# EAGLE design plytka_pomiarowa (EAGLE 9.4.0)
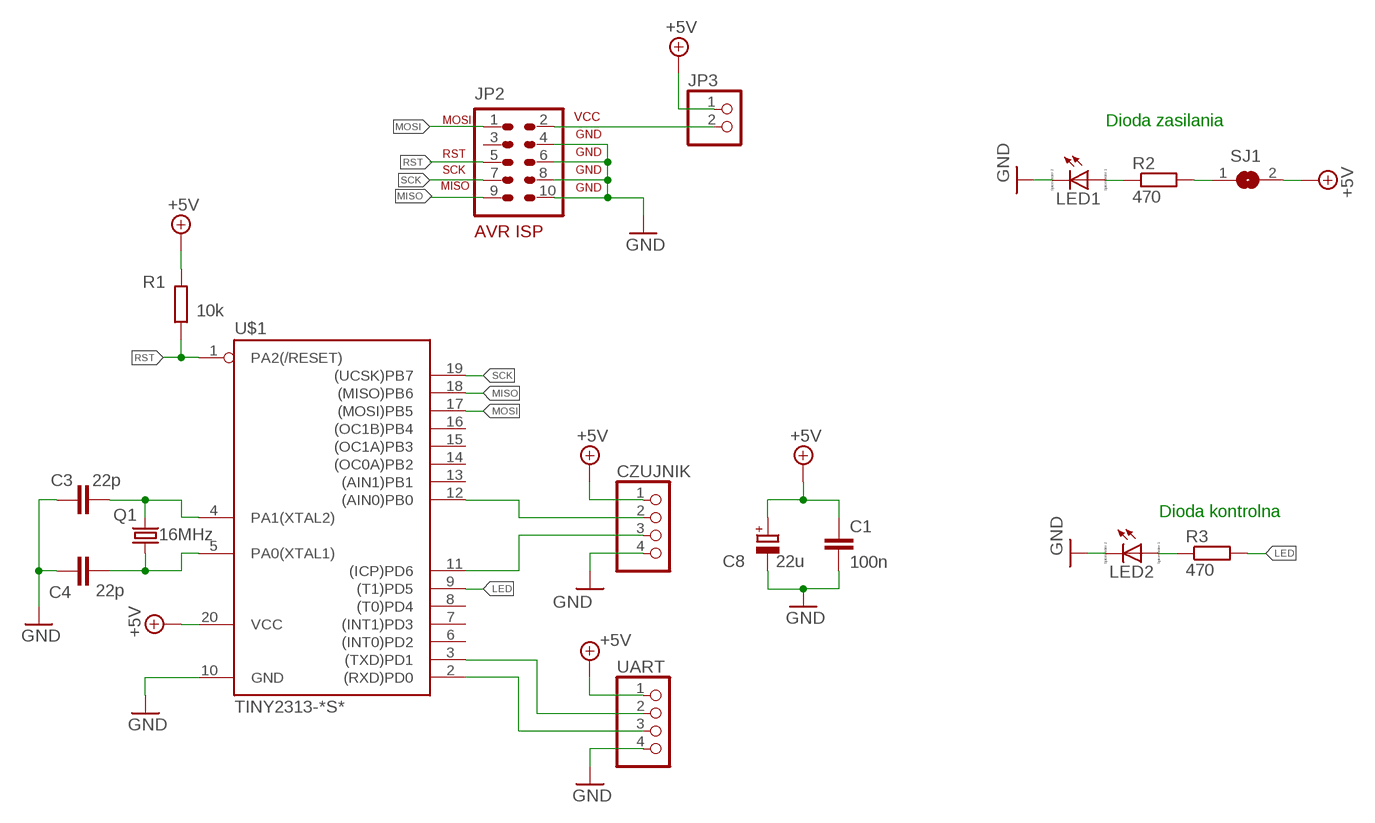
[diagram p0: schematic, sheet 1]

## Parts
C1  100n  C-EUC1206  [C1206]
C3  22p  C-EUC1206  [C1206]
C4  22p  C-EUC1206  [C1206]
C8  22u  CPOL-EUSMCB  [SMC_B]
CZUJNIK  PINHD-1X4  [1X04]
JP2  AVR-ISP-10  [AVR-ISP-10]
JP3  PINHD-1X2  [1X02]
LED1  LED_E  [LED_1206]
LED2  LED_E  [LED_1206]
Q1  16MHz  KX-KS  [11.4X4.5]
R1  10k  R-EU_M1206  [M1206]
R2  470  R-EU_M1206  [M1206]
R3  470  R-EU_M1206  [M1206]
SJ1  SJ  [SJ]
U$1  TINY2313-*S*  [SO20L$]
UART  PINHD-1X4  [1X04]

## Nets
+5V: C1.1 C8.+ CZUJNIK.1 JP3.1 R1.2 SJ1.2 U$1.20(VCC) UART.1
ECHO: CZUJNIK.3 U$1.11((ICP)PD6)
GND: C1.2 C3.1 C4.1 C8.- CZUJNIK.4 JP2.4 JP2.6 JP2.8 JP2.10 LED1.C LED2.C U$1.10(GND) UART.4
LED: R3.2 U$1.9((T1)PD5)
MISO: JP2.9 U$1.18((MISO)PB6)
MOSI: JP2.1 U$1.17((MOSI)PB5)
N$1: C3.2 Q1.2 U$1.4(PA1(XTAL2))
N$2: C4.2 Q1.1 U$1.5(PA0(XTAL1))
N$3: JP2.2 JP3.2
N$4: R2.2 SJ1.1
N$5: LED1.A R2.1
N$7: LED2.A R3.1
RST: JP2.5 R1.1 U$1.1(PA2(/RESET))
RX: U$1.2((RXD)PD0) UART.3
SCK: JP2.7 U$1.19((UCSK)PB7)
TRIG: CZUJNIK.2 U$1.12((AIN0)PB0)
TX: U$1.3((TXD)PD1) UART.2
Unconnected: JP2.3 U$1.6((INT0)PD2) U$1.7((INT1)PD3) U$1.8((T0)PD4) U$1.13((AIN1)PB1) U$1.14((OC0A)PB2) U$1.15((OC1A)PB3) U$1.16((OC1B)PB4)

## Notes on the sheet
- Dioda zasilania
- Dioda kontrolna

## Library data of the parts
C1 C3 C4 = resistor:C-EU: CAPACITOR, European symbol
C8 = resistor:CPOL-EU: POLARIZED CAPACITOR, European symbol
CZUJNIK = pinhead:PINHD-1X4: PIN HEADER
JP2 = avr-7:AVR-ISP-10: AVR ISP-10 Serial Programming Header
JP3 = pinhead:PINHD-1X2: PIN HEADER
LED1 LED2 = eagle-ltspice:LED_E: LED; SPICEMODEL: NONE; SPICEPREFIX: D; SPICETYPE: diode
Q1 = crystal-geyer_V1_0:KX
R1-R3 = resistor:R-EU_: RESISTOR, European symbol
SJ1 = jumper:SJ: SMD solder JUMPER
U$1 = avr-7:TINY2313*: Atmel Tiny2313 2K Flash, 128 bytes EEPROM, 128 bytes RAM
UART = pinhead:PINHD-1X4: PIN HEADER; SPICEPREFIX: E

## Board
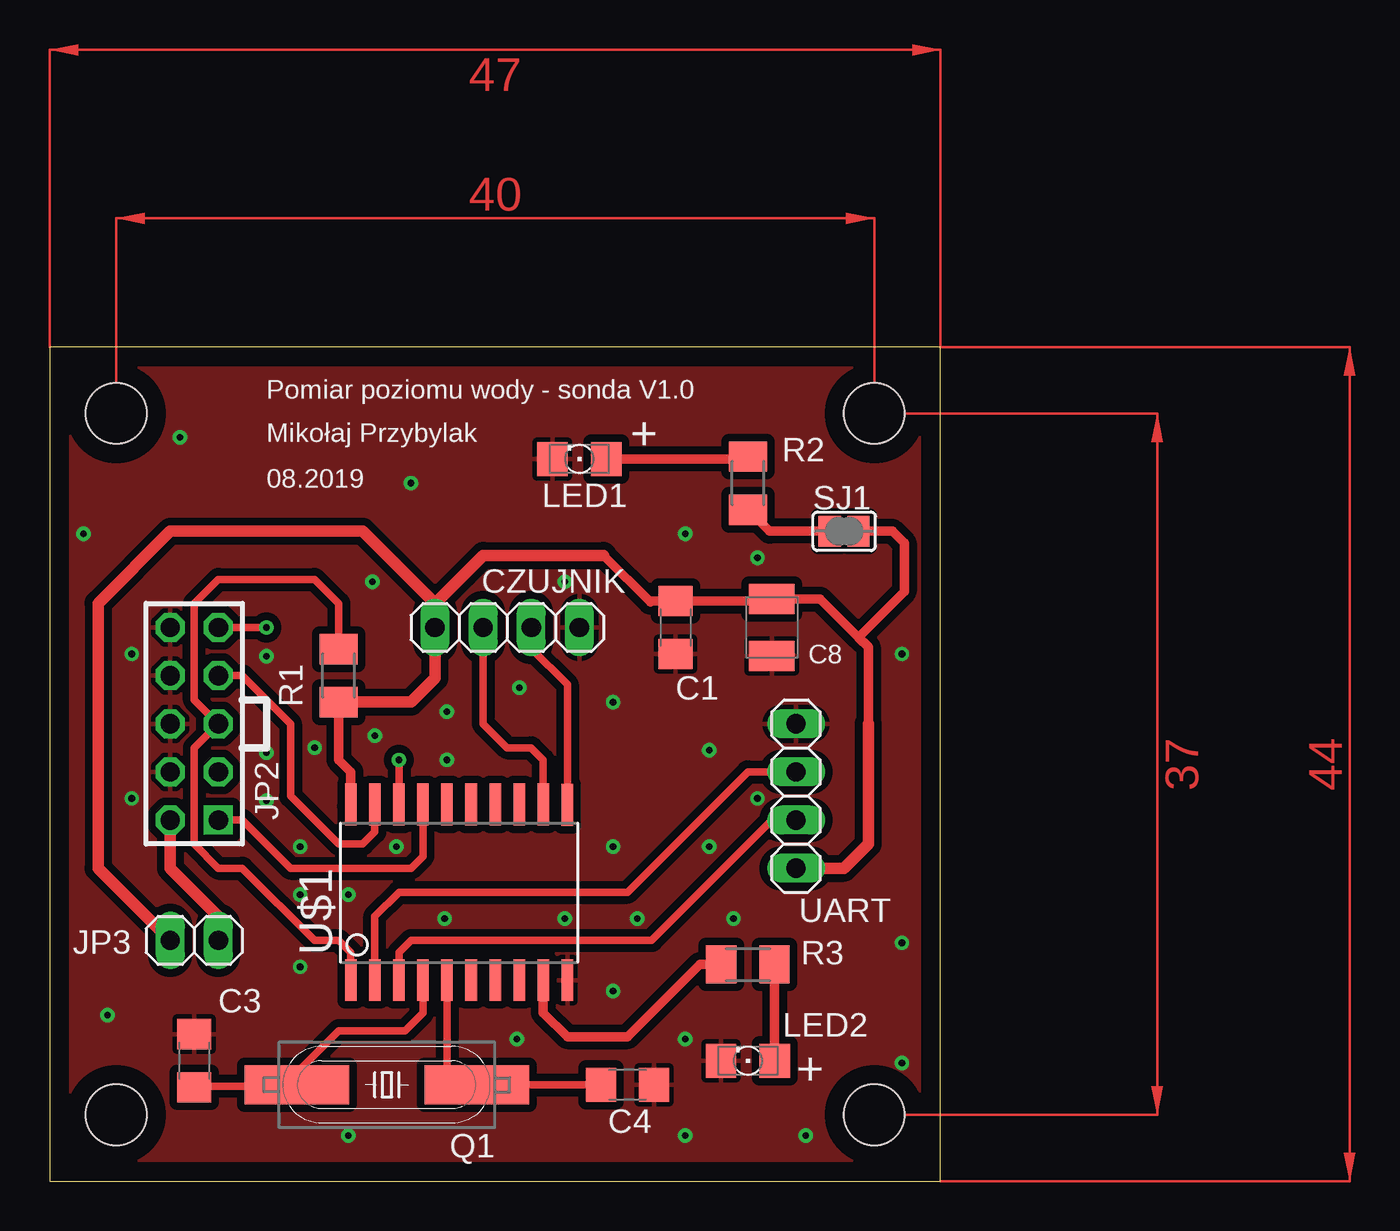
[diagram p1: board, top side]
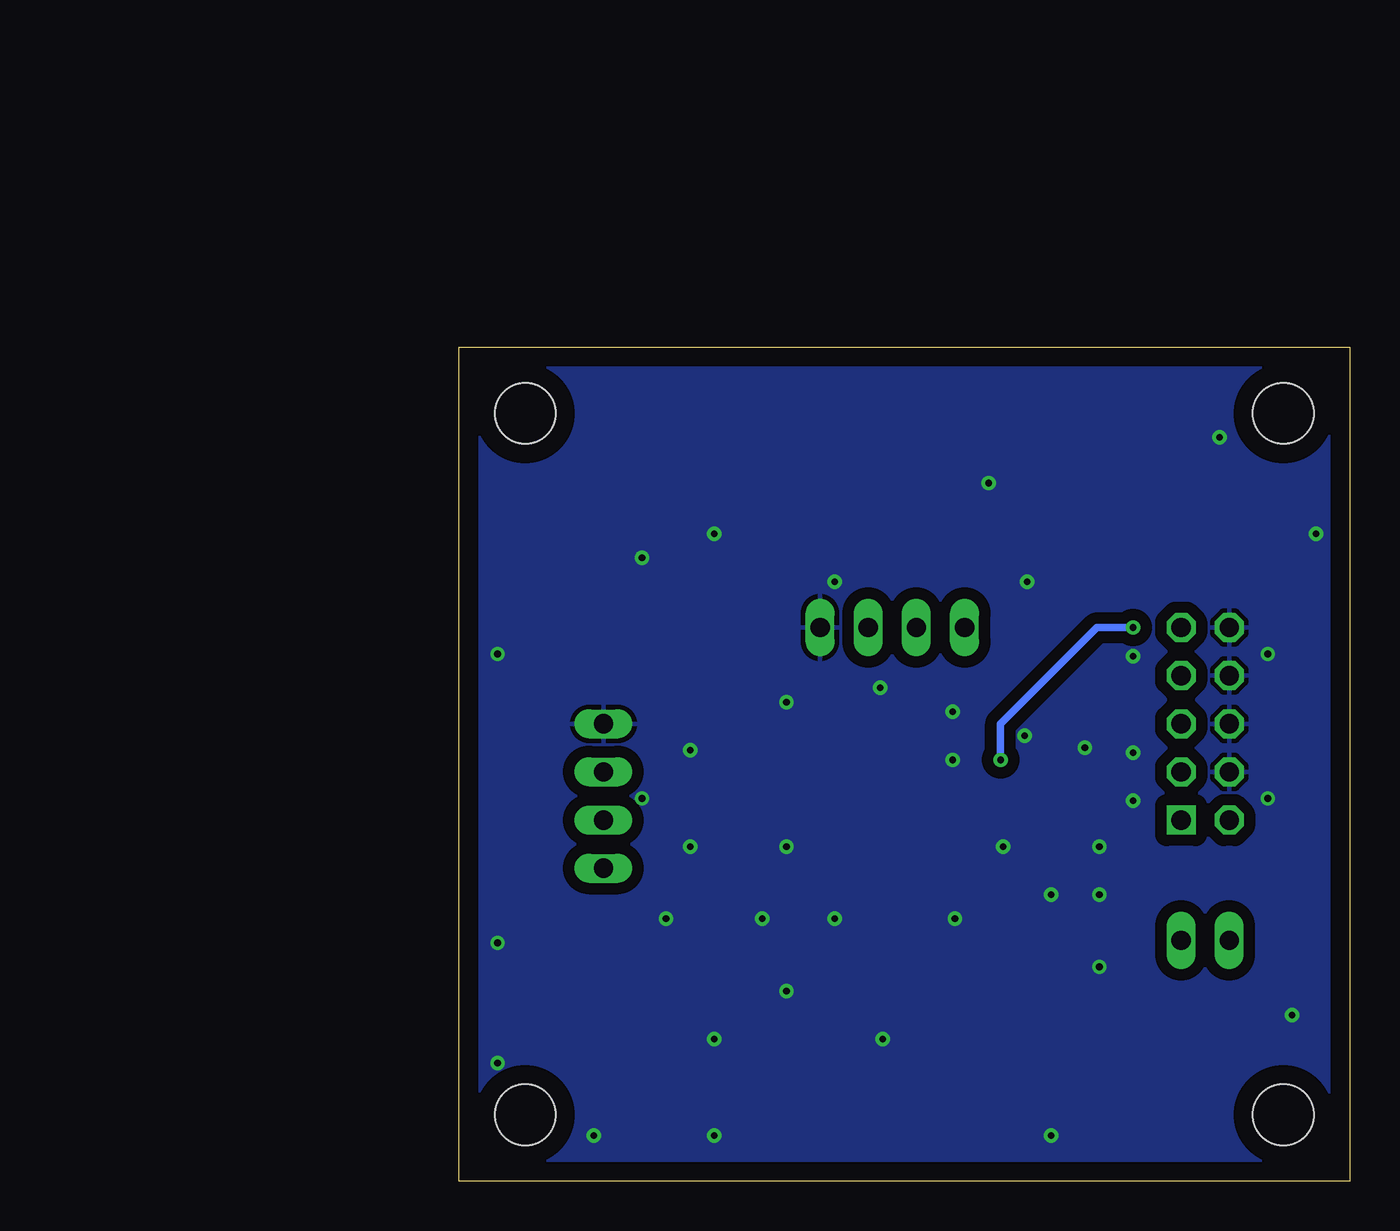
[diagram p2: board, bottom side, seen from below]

Size 47 x 44 mm. Coordinates in mm from the lower left corner, seen from the top.
Outline: 0,0 47,0 47,44 0,44 0,0
Copper layers (1*16): Top 0.035mm / dielectric 1.5mm / Bottom 0.035mm
Design rules "default *": minimum track width 6mil, minimum drill 0.5mm, track to track 10mil, track to pad 10mil, pad to pad 10mil, via to via 10mil, smd to smd 6mil, copper to edge 40mil, drill to drill 6mil, minimum pad ring 10mil, minimum via ring 8mil, stop-mask expansion 4mil, vias tented up to drill 0mil, thermal gap 10mil
Holes 3.2 mm at 3.5,40.5 43.5,40.5 43.5,3.5 3.5,3.5

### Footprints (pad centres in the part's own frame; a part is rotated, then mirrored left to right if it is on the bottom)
C1206 = smd 1.6 x 1.8: 1 -1.4,0; 2 1.4,0
SMC_B = smd 1.6 x 2.4: + -1.5,0; - 1.5,0
1X04 = drill 1.016 long: 1 -3.81,0; 2 -1.27,0; 3 1.27,0; 4 3.81,0
AVR-ISP-10 = drill 1.016 square: 1 -5.08,-1.27 | drill 1.016 octagon: 2 -5.08,1.27; 3 -2.54,-1.27; 4 -2.54,1.27; 5 0,-1.27; 6 0,1.27; 7 2.54,-1.27; 8 2.54,1.27; 9 5.08,-1.27; 10 5.08,1.27
1X02 = drill 1.016 long: 1 -1.27,0; 2 1.27,0
LED_1206 = smd 1.6 x 1.803: A -1.422,0; C 1.422,0
11.4X4.5 = smd 5.5 x 2.08: 1 -4.75,0; 2 4.75,0
M1206 = smd 1.6 x 2: 1 -1.4,0; 2 1.4,0
SJ = smd 1.168 x 1.6: 1 -0.762,0; 2 0.762,0
SO20L$ = smd 0.61 x 2.21: 1 -5.715,-4.636; 2 -4.445,-4.636; 3 -3.175,-4.636; 4 -1.905,-4.636; 5 -0.635,-4.636; 6 0.635,-4.636; 7 1.905,-4.636; 8 3.175,-4.636; 9 4.445,-4.636; 10 5.715,-4.636; 11 5.715,4.61; 12 4.445,4.636; 13 3.175,4.636; 14 1.905,4.636; 15 0.635,4.636; 16 -0.635,4.636; 17 -1.905,4.636; 18 -3.175,4.636; 19 -4.445,4.636; 20 -5.715,4.636

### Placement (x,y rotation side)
C1  33.02,29.21 270 top
C3  7.62,6.35 270 top
C4  30.48,5.08 180 top
C8  38.1,29.21 270 top
CZUJNIK  24.13,29.21 0 top
JP2  7.62,24.13 90 top
JP3  7.62,12.7 0 top
LED1  27.94,38.1 180 top
LED2  36.83,6.35 180 top
Q1  17.78,5.08 180 top
R1  15.24,26.67 270 top
R2  36.83,36.83 270 top
R3  36.83,11.43 180 top
SJ1  41.91,34.29 0 top
U$1  21.59,15.24 0 top
UART  39.37,20.32 90 top

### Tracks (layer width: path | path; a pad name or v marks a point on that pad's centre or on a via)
+5V
  Top 0.508: 29.21,33.02 31.68,30.55 31.75,30.61 C1.1 38,30.61 C8.+ 40.64,30.71 42.66,28.69 | 42.66,28.69 43.18,28.17 43.18,24.13 | SJ1.2 44.45,34.29 45.09,33.66 45.09,31.11 42.66,28.69 | U$1.20 15.88,21.59 15.24,22.23 R1.2
  Top 0.61: 15.88,19.68 U$1.20 | 20.32,27.94 CZUJNIK.1 | CZUJNIK.1 20.32,30.48 | 20.32,30.48 22.86,33.02 29.21,33.02 | UART.1 41.91,16.51 43.18,17.78 43.18,24.13 | R1.2 19.05,25.27 20.32,26.54 CZUJNIK.1 | 20.32,30.48 16.51,34.29 6.35,34.29 2.54,30.48 2.54,16.51 JP3.1
ECHO
  Top 0.406: CZUJNIK.3 25.4,28.11 27.3,26.2 U$1.11
GND  (via drill 0.35)
  other vias: 19.05,36.83 13.97,22.86 11.43,27.69 11.43,22.61 11.43,20.07 13.21,17.65 18.29,17.65 20.83,13.84 27.18,13.84 30.99,13.84 34.8,17.65 37.34,20.19 29.72,25.27 34.8,22.73 36.07,13.84 44.96,12.57 44.96,6.22 39.88,2.41 24.64,7.49 29.72,17.65 33.53,7.49 3.05,8.76 13.21,11.3 4.32,20.19 4.32,27.81 1.78,34.16 6.86,39.24 17.02,31.62 27.18,31.62 33.53,34.16 37.34,32.89 44.96,27.81 33.53,2.41 15.75,2.41 13.21,15.11 15.75,15.11 17.14,23.5 20.95,22.23 20.95,24.77 24.77,26.04 29.72,10.03
  pour Top (isolate 0.406): -2.54,45.72 49.53,45.72 49.53,-1.27 -2.54,-1.27
  pour Bottom (isolate 0.61): -1.27,45.72 49.53,45.72 49.53,-3.81 -1.27,-3.81
LED
  Top 0.508: U$1.9 26.04,8.89 27.3,7.62 30.48,7.62 34.29,11.43 R3.2
MISO  (via drill 0.35)
  Top 0.406: JP2.9 v11.43,29.21 | 18.41,20.57 U$1.18 v18.41,22.23
  Bottom 0.406: v18.41,22.23 18.41,24.13 13.34,29.21 v11.43,29.21
MOSI
  Top 0.406: JP2.1 10.16,19.05 12.7,16.51 19.05,16.51 19.68,17.14 U$1.17
N$1
  Top 0.406: C3.2 7.66,4.99 12.94,4.99 Q1.2 | U$1.4 19.68,8.89 18.73,7.94 15.24,7.94 12.7,5.4 12.7,5.08
  Top 0.508: Q1.2 12.71,5.08 12.7,5.08
N$2
  Top 0.406: U$1.5 20.95,5.08 Q1.1 C4.2
N$3
  Top 0.61: JP2.2 6.35,16.51 8.89,13.97 JP3.2
N$4
  Top 0.508: SJ1.1 37.97,34.29 R2.2
N$5
  Top 0.508: R2.1 36.7,38.1 LED1.A
N$7
  Top 0.508: R3.1 38.23,6.37 LED2.A
RST
  Top 0.406: U$1.1 15.88,12.06 15.24,12.7 13.97,12.7 10.16,16.51 8.89,16.51 7.62,17.78 7.62,22.86 JP2.5 7.62,25.4 7.62,30.48 8.89,31.75 13.97,31.75 15.24,30.48 R1.1
RX
  Top 0.406: UART.3 36.83,21.59 30.48,15.24 18.41,15.24 17.14,13.97 U$1.2
SCK
  Top 0.406: JP2.7 10.16,26.67 12.7,24.13 12.7,20.32 15.24,17.78 16.51,17.78 17.14,18.41 U$1.19
TRIG
  Top 0.406: CZUJNIK.2 22.86,24.13 24.13,22.86 25.4,22.86 26.04,22.23 U$1.12
TX
  Top 0.406: UART.2 38.1,19.05 31.75,12.7 19.05,12.7 18.41,12.06 U$1.3
(copper drawn outside any net)
  shapes: Top area x4

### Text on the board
tPlace: Pomiar poziomu wody - sonda V1.0 | Mikołaj Przybylak | + | 08.2019 | +

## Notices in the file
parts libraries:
crystal-geyer_V1_0: Copyright: Geyer-Electronic
